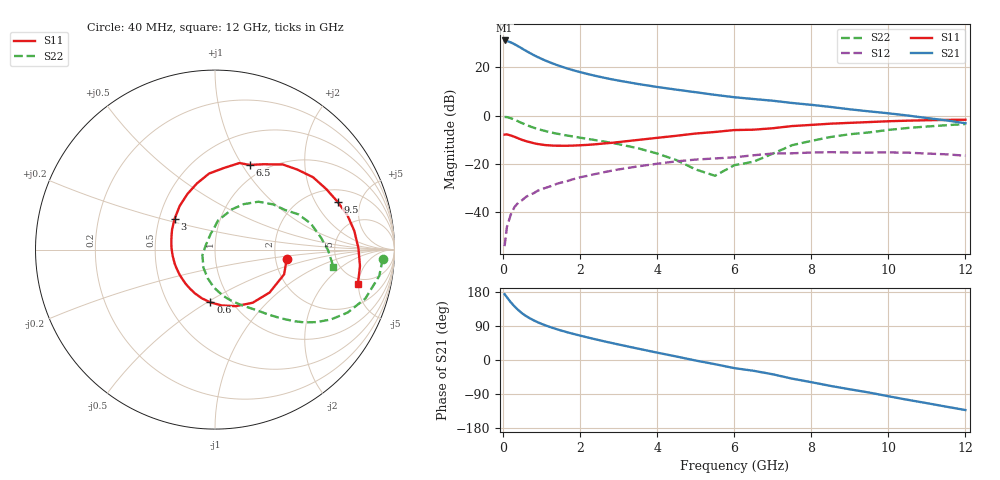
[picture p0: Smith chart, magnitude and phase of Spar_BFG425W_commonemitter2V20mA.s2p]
! Filename: 220bfg425.001
! BFG425W Field C1
! V1=8.621E-001V,V2=2.000E+000V, I1=2.817E-004A, I2=2.003E-002A
# GHz  S  MA  R 50
!  S11  S21  S12  S22
!Freq(GHz)  Mag  Ang  Mag  Ang  Mag  Ang  Mag  Ang
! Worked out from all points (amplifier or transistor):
!   44 points, 40 MHz to 12 GHz, reference 50 ohm
!   highest |S21| = 31.0 dB at 40 MHz (marker M1)
!   |S21| within 3 dB of that: start of sweep to 456.7 MHz
!   unconditionally stable (mu >= 1): 1.275 GHz to end of sweep
!   at 700 MHz: K = 0.76, MSG = 29.3 dB, |S12| = -32.8 dB
!   at 2.4 GHz: K = 1.16, MAG = 17.8 dB, |S12| = -24.2 dB
!   at 12 GHz: K = 1.35, MAG = 3.2 dB, |S12| = -16.6 dB
!   lowest NFmin = 1.90 dB at 900 GHz
!   S11 on the Smith chart (normalised r, x): 40 MHz: 2.30, -0.30; 600 MHz: 0.80, -0.52; 3 GHz: 0.60, +0.22; 6.5 GHz: 0.85, +1.08; 9.5 GHz: 2.69, +3.11; 12 GHz: 4.18, -4.89
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0.04  0.403 -7.7  35.57 173.7  0.002 74.2  0.936 -3.1
0.1  0.409 -19.6  34.63 165.5  0.005 83.8  0.927 -9.1
0.2  0.387 -38.1  32.48 152.3  0.009 76.2  0.881 -18.0
0.3  0.363 -54.6  29.67 141.1  0.013 71.5  0.818 -25.4
0.4  0.336 -69.8  26.76 131.3  0.016 67.9  0.753 -31.2
0.5  0.313 -83.4  24.04 122.7  0.018 64.7  0.693 -35.7
0.6  0.295 -95.0  21.59 115.7  0.021 62.9  0.642 -39.2
0.7  0.281 -105.2  19.49 109.8  0.023 61.4  0.597 -42.0
0.8  0.268 -114.8  17.69 104.4  0.025 60.5  0.559 -44.3
0.9  0.258 -123.0  16.15 99.6  0.028 59.7  0.528 -46.3
1  0.251 -130.7  14.82 95.3  0.03 59.0  0.501 -48.1
1.2  0.242 -144.0  12.68 87.7  0.034 57.7  0.457 -51.4
1.6  0.237 -165.9  9.759 75.1  0.043 54.7  0.394 -57.3
2.2  0.248 169.0  7.187 59.4  0.057 49.1  0.329 -66.7
3  0.283 142.7  5.268 40.9  0.077 39.5  0.256 -81.1
4.5  0.382 105.3  3.425 9.2  0.113 17.7  0.12 -122.4
5.5  0.457 83.9  2.675 -11.0  0.13 1.9  0.057 153.6
6.5  0.51 67.6  2.193 -28.4  0.151 -10.5  0.111 95.0
8.5  0.679 36.4  1.505 -68.4  0.175 -47.3  0.36 47.8
9.5  0.733 21.3  1.219 -85.8  0.172 -63.8  0.448 29.6
10.5  0.783 7.7  1.002 -105.0  0.171 -82.2  0.553 15.3
12  0.819 -13.6  0.693 -132.0  0.148 -111.6  0.667 -8.4
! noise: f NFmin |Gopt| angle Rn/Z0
900  1.9  0.19  -165.5  0.18
2000  2.2  0.17  -155.5  0.2
